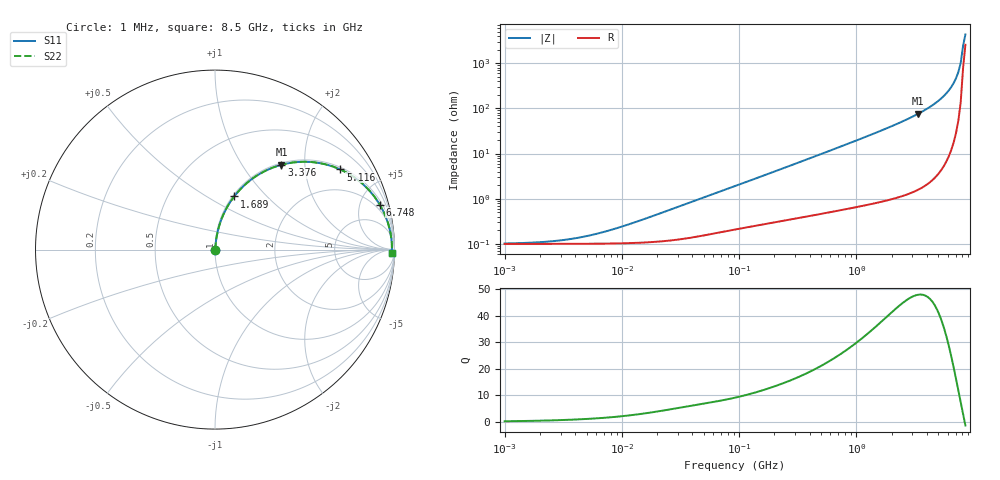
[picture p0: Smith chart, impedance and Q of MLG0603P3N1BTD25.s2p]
! S-Parameter Data Generated by TDK Corporation
! Copyright(C) 2025 TDK Corporation.
! All Rights Reserved.
! TDK P/N: MLG0603P3N1BTD25 (SMD / SMT Inductor (Coil))
! Property: L=3.1nH at 500MHz
! Size(LxWxT): 0.6x0.3x0.3mm
! Model Type: s2p (Touchstone File Format Version 1.0)
! Frequency: DC=Yes Start=1MHz Stop=8500MHz 198points Log-sweep
! Model Generated on Feb. 6, 2025
! Terms and conditions regarding TDK Simulation Models:
! 1)This simulation model is being provided solely for informational
!  purposes. Please refer to the specifications of the products in
!  terms of detailed characteristics of such products.
! 2)In no event shall TDK Corporation of any of its subsidiaries be
!  liable for any loss or damage arising, directly or indirectly,
!  from any information contained in this simulation model, including,
!  but not limited to loss or damages arising from any inaccuracies,
!  omissions or errors in connection with such information.
! 3)Any and all copyrights on this simulation model are owned by
!  TDK Corporation.  Duplication or redistribution of this simulation
!  model without prior written permission from TDK Corporation
!  is prohibited.
! 4)This simulation model is subject to any modification or change
!  without any prior notice.
! 5)Neither TDK Corporation nor any of its subsidiaries shall make any
!  warranty, express or implied, including but not limited to the
!  correctness, implied warranties of merchantability and fitness for
!  a particular purpose with respect to this simulation models.
! 6)The use of this simulation model shall be deemed to have consented
!  to the terms and conditions hereof.
! Port Assignments:
!  1 ---@@@--- 2
! Applicable Conditions:
!  Temperature = 25 degC
!  DC Bias Current = 0 A
!  Small Signal Operation
# Hz S MA R 50
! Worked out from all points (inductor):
!   197 points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, 1 MHz to 8.5 GHz, reference 50 ohm
!   read as one part in series: L = 3.47 nH near 15.23 MHz
!   highest Q = 47.9 at 3.376 GHz (marker M1), where L = 3.59 nH
!   self-resonance near 8.117 GHz
!   S11 on the Smith chart (normalised r, x): 1 MHz: 1.00, +0.00; 1.689 GHz: 1.02, +0.67; 3.376 GHz: 1.03, +1.52; 5.116 GHz: 1.08, +3.07; 6.748 GHz: 1.35, +7.22; 8.5 GHz: 52, -69
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1000000  0.001023 12.4  0.999 -0.0  0.999 -0.0  0.001023 12.4
2403882  0.001131 27.7  0.999 -0.0  0.999 -0.0  0.001131 27.7
4587603  0.001422 44.9  0.999 -0.1  0.999 -0.1  0.001422 44.9
8755050  0.002171 61.8  0.999 -0.1  0.999 -0.1  0.002171 61.8
2.10461e7  0.00471 75.9  0.9989 -0.3  0.9989 -0.3  0.00471 75.9
9.219544e7  0.01904 82.6  0.9977 -1.1  0.9977 -1.1  0.01904 82.6
4.229561e8  0.0821 82.3  0.9924 -4.7  0.9924 -4.7  0.0821 82.3
8.852465e8  0.1684 78.3  0.9797 -9.7  0.9797 -9.7  0.1684 78.3
1.689417e9  0.3152 70.1  0.9409 -18.4  0.9409 -18.4  0.3152 70.1
1.940355e9  0.3599 67.5  0.9242 -21.1  0.9242 -21.1  0.3599 67.5
2.559585e9  0.4672 60.9  0.8739 -27.8  0.8739 -27.8  0.4672 60.9
3.37643e9  0.6 51.9  0.7876 -36.9  0.7876 -36.9  0.6 51.9
4.253027e9  0.7263 42.2  0.6718 -46.6  0.6718 -46.6  0.7263 42.2
5.115526e9  0.8289 32.6  0.5391 -56.0  0.5391 -56.0  0.8289 32.6
5.87536e9  0.8982 24.3  0.4124 -63.9  0.4124 -63.9  0.8982 24.3
6.44363e9  0.9363 18.4  0.3152 -69.3  0.3152 -69.3  0.9363 18.4
6.748056e9  0.952 15.2  0.2632 -72.0  0.2632 -72.0  0.952 15.2
7.066863e9  0.9651 12.1  0.2094 -74.4  0.2094 -74.4  0.9651 12.1
7.400733e9  0.9752 8.8  0.154 -76.3  0.154 -76.3  0.9752 8.8
7.750377e9  0.9822 5.6  0.09768 -76.7  0.09768 -76.7  0.9822 5.6
8.116539e9  0.9859 2.3  0.04152 -69.0  0.04152 -69.0  0.9859 2.3
8.5e9  0.9862 -1.1  0.0229 52.6  0.0229 52.6  0.9862 -1.1
